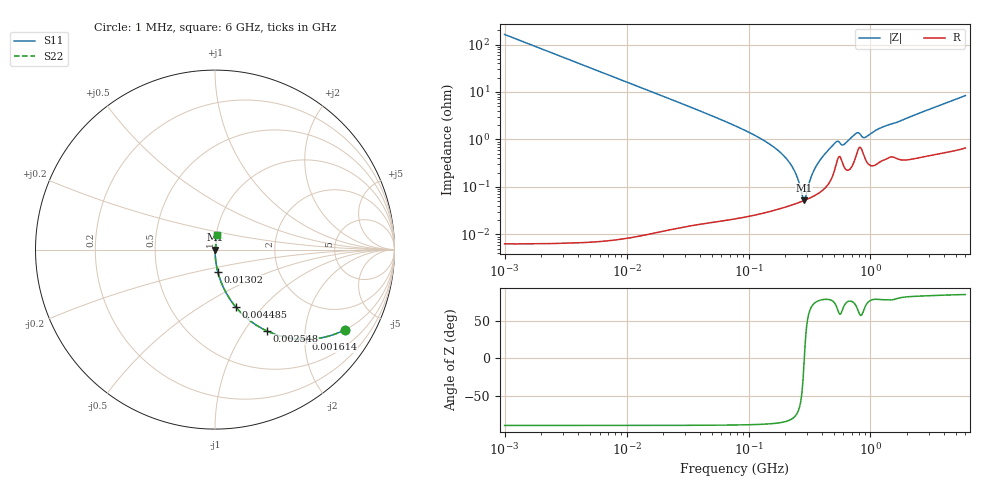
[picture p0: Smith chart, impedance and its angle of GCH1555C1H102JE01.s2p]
!Murata Part Number: GCH1555C1H102JE01
!These Parameters are Measured in Series Mode Connection
!Data Generated on Jun 19, 2026
!  o--ll--o
!Port1  Port2
!  o------o
!Operation Temp=25[degC], DC Bias Voltage=0[V]
!Freq. Start=1000[kHz] Stop=6[GHz] 401[Steps]
# Hz S RI R 50
!Freq.(Hz) S11(Real) S11(Imag) S21(Real) S21(Imag) S12(Real) S12(Imag) S22(Real) S22(Imag)
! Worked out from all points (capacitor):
!   401 points, 1 MHz to 6 GHz, reference 50 ohm
!   read as one part in series: C = 977 pF near 1.044 MHz
!   lowest |Z| = 51.7 mohm at 285.6 MHz (marker M1)
!   series resonance near 286.6 MHz, so ESL is about 320 pH
!   S11 on the Smith chart (normalised r, x): 1 MHz: 1.00, -3.26; 1.614 MHz: 1.00, -2.02; 2.548 MHz: 1.00, -1.28; 4.485 MHz: 1.00, -0.73; 13.02 MHz: 1.00, -0.25; 6 GHz: 1.01, +0.17
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1000000  0.7262 -0.4459  0.2738 0.4459  0.2738 0.4459  0.7262 -0.4459
1613609  0.5046 -0.4999  0.4954 0.4999  0.4954 0.4999  0.5046 -0.4999
2547717  0.2901 -0.4537  0.7099 0.4537  0.7099 0.4537  0.2901 -0.4537
4293785  0.1258 -0.3315  0.8742 0.3315  0.8742 0.3315  0.1258 -0.3315
4484676  0.1165 -0.3207  0.8835 0.3207  0.8835 0.3207  0.1165 -0.3207
1.301831e7  0.0154 -0.1229  0.9846 0.1229  0.9846 0.1229  0.0154 -0.1229
1.843659e7  0.00778 -0.0872  0.9922 0.0872  0.9922 0.0872  0.00778 -0.0872
7.745967e7  0.000589 -0.0194  0.9994 0.0194  0.9994 0.0194  0.000589 -0.0194
1.363501e8  0.00037 -0.00921  0.9996 0.00921  0.9996 0.00921  0.00037 -0.00921
1.930997e8  0.000385 -0.0046  0.9996 0.0046  0.9996 0.0046  0.000385 -0.0046
2.348496e8  0.000433 -0.00229  0.9996 0.00229  0.9996 0.00229  0.000433 -0.00229
2.734687e8  0.000493 -0.00054  0.9995 0.00054  0.9995 0.00054  0.000493 -0.00054
2.856264e8  0.000516 -4.06e-05  0.9995 4.06e-05  0.9995 4.06e-05  0.000516 -4.06e-05
2.983246e8  0.00054 0.000461  0.9995 -0.000461  0.9995 -0.000461  0.00054 0.000461
3.325952e8  0.000618 0.00174  0.9994 -0.00174  0.9994 -0.00174  0.000618 0.00174
3.872876e8  0.000788 0.00363  0.9992 -0.00363  0.9992 -0.00363  0.000788 0.00363
5.138348e8  0.00257 0.00812  0.9974 -0.00812  0.9974 -0.00812  0.00257 0.00812
6.11486e8  0.00261 0.0075  0.9974 -0.0075  0.9974 -0.0075  0.00261 0.0075
7.767579e8  0.00544 0.0126  0.9946 -0.0126  0.9946 -0.0126  0.00544 0.0126
9.044891e8  0.00401 0.0102  0.996 -0.0102  0.996 -0.0102  0.00401 0.0102
1.428092e9  0.00457 0.02  0.9954 -0.02  0.9954 -0.02  0.00457 0.02
6e9  0.0133 0.082  0.9867 -0.082  0.9867 -0.082  0.0133 0.082
